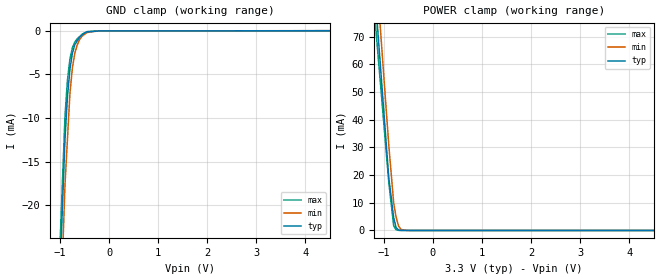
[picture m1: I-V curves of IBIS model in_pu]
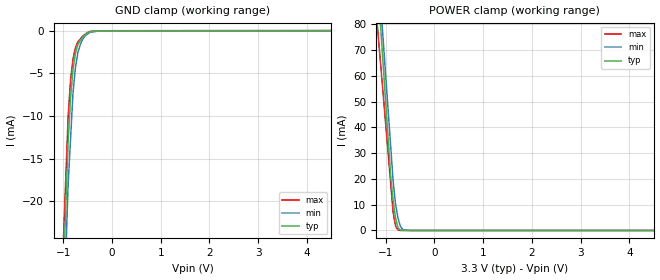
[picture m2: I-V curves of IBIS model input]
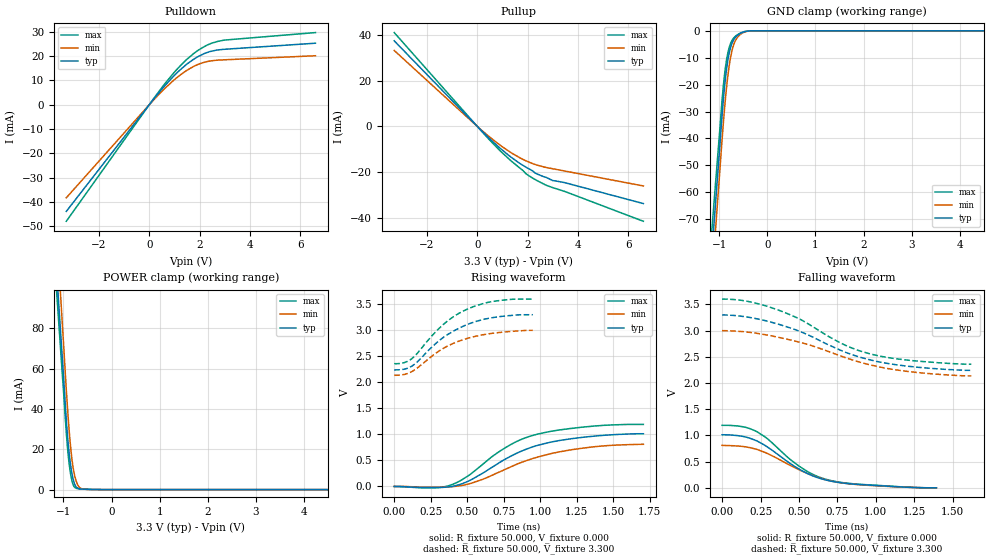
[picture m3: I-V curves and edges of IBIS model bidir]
|Texas Instruments Incorporated
|118dB SNR Stereo Audio ADC
[IBIS Ver]   4.0
[File Name] pcm4202.ibs
[File Rev] 3.0
[Date]   10-06-2009
[Notes]  Quality Check of this IBIS model: Model Passes IBIS Check. Model
   parses into ICX IS. Simulates with Hyperlynx.
   1. MIN TYP MAX information is based on Temperature and Voltage
   characteristics only.
   2. Package information extracted using Tektronix IConnect Software.
[Source]   Texas Instruments Incorporated.
   Analog-eLab, HPA
   12500 TI Blvd
   Dallas, TX -75243
   For Support e-mail: elab_ibis@list.ti.com
[Disclaimer]
| This model is designed as an aid for customers of Texas Instruments.
| TI and its licensors and suppliers make no warranties, either expressed
| or implied, with respect to this  model, including the warranties of
| merchantability or fitness for a particular purpose. The model is
| provided solely on an "as is" basis. The entire risk as to its quality
| and performance is with the customer.
[Copyright]
| (C) Copyright 2011 Texas Instruments Incorporated. All rights reserved.
[Component] PCM4202
[Manufacturer] TI
[Package]
| variable   typ   min   max
R_pkg  1.000E-02   1.000E-02   1.000E-02
L_pkg  2.970E-09   2.790E-09   3.150E-09
C_pkg  4.580E-13   1.880E-13   7.280E-13
[Pin] signal_name  model_name  R_pin  L_pin C_pin
1   VREFL   term   1.000E-02   3.150E-09   7.280E-13
2   AGNDL   GND   1.000E-02   3.090E-09   6.380E-13
3   VCOML   POWER   1.000E-02   3.030E-09   5.480E-13
4   VINL_P   term   1.000E-02   2.970E-09   4.580E-13
5   VINL_M   term   1.000E-02   2.910E-09   3.680E-13
6   FMT0   input   1.000E-02   2.850E-09   2.780E-13
7   FMT1   input   1.000E-02   2.790E-09   1.880E-13
8   S/*M   input   1.000E-02   2.790E-09   1.880E-13
9   OSR0   input   1.000E-02   2.850E-09   2.780E-13
10  OSR1   input   1.000E-02   2.910E-09   3.680E-13
11  OSR2   input   1.000E-02   2.970E-09   4.580E-13
12  BYPAS   input   1.000E-02   3.030E-09   5.480E-13
13  DGND   GND   1.000E-02   3.090E-09   6.380E-13
14  VDD   POWER   1.000E-02   3.150E-09   7.280E-13
15  DATA/DSDR   output  1.000E-02   3.150E-09   7.280E-13
16  BCK/DSDL   bidir   1.000E-02   3.090E-09   6.380E-13
17  LRCK/DSDBCK bidir   1.000E-02   3.030E-09   5.480E-13
18  SCKI   input   1.000E-02   2.970E-09   4.580E-13
19  *RST   in_pu   1.000E-02   2.910E-09   3.680E-13
20  CLIPR   output  1.000E-02   2.850E-09   2.780E-13
21  CLIPL   output  1.000E-02   2.790E-09   1.880E-13
22  VCC   POWER   1.000E-02   2.790E-09   1.880E-13
23  AGND   GND   1.000E-02   2.850E-09   2.780E-13
24  VINR_M   term   1.000E-02   2.910E-09   3.680E-13
25  VINR_P   term   1.000E-02   2.970E-09   4.580E-13
26  VCOMR   POWER   1.000E-02   3.030E-09   5.480E-13
27  AGNDR   GND   1.000E-02   3.090E-09   6.380E-13
28  VREFR   term   1.000E-02   3.150E-09   7.280E-13
[Diff Pin] inv_pin vdiff tdelay_typ tdelay_min tdelay_max
4  5   NA   NA  NA  NA
25 24  NA   NA  NA  NA
[Model]  term
Model_type Terminator
C_comp   0   0   0
[Voltage Range]  5.00  4.75  5.25
[Temperature Range] 25   70   -10
| Models and submodels in the file (5): in_pu (Input), input (Input), bidir (I/O), output (Output), term (Terminator)
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[Model] in_pu
Model_type Input
Vinl = 990.000mV
Vinh = 2.31000V
C_comp 886.000fF 877.000fF 891.000fF
| variable typ   min   max
[Voltage Range] 3.30000V 3.00000V 3.60000V
[POWER Clamp Reference] 3.30000V 3.00000V 3.60000V
[GND Clamp Reference] 0.00000V 0.00000V 0.00000V
[Temperature Range] 25   70   -10
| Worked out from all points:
|   GND clamp passes 1 mA (typ) near -0.63 V on its own axis
|   POWER clamp passes 1 mA (typ) near -0.75 V on its own axis
[GND Clamp]
-3.3V     -369.9mA   -412.4mA   -356.3mA
-900mV    -12.43mA   -17.61mA   -9.82mA
-850mV    -7.567mA   -12.41mA   -5.659mA
-800mV    -4.432mA   -7.205mA   -3.254mA
-750mV    -2.598mA   -4.295mA   -1.972mA
-700mV    -1.601mA   -2.555mA   -1.295mA
-650mV    -1.153mA   -1.615mA   -919.1uA
-600mV    -704.6uA   -986.7uA   -654.8uA
-550mV    -481.7uA   -601.4uA   -390.5uA
-450mV    -126.3uA   -189.9uA   -94.7uA
-225mV    -21.91uA   -16.78uA   -19.72uA
6.6V      22.46uA    24.13uA    17.33uA
[POWER Clamp]
-3.3V     589.8mA    621.3mA    521.2mA
-1.15V    78.61mA    92.45mA    70.07mA
-1.1V     66.72mA    80.15mA    59.58mA
-1.05V    54.83mA    67.86mA    49.09mA
-900mV    19.17mA    30.96mA    17.62mA
-800mV    4.66mA     10.03mA    1.697mA
-750mV    1.031mA    4.804mA    243.3uA
-700mV    165.1uA    1.618mA    31.19uA
-650mV    23.84uA    330.3uA    28.07uA
-550mV    16.51uA    39.34uA    21.83uA
6.6V      0A         0A         0A
[Model] input
Model_type Input
Vinl = 990.000mV
Vinh = 2.31000V
C_comp 696.000fF 674.000fF 706.000fF
| variable typ   min   max
[Voltage Range] 3.30000V 3.00000V 3.60000V
[POWER Clamp Reference] 3.30000V 3.00000V 3.60000V
[GND Clamp Reference] 0.00000V 0.00000V 0.00000V
[Temperature Range] 25   70   -10
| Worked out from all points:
|   GND clamp passes 1 mA (typ) near -0.63 V on its own axis
|   POWER clamp passes 1 mA (typ) near -0.75 V on its own axis
[GND Clamp]
-3.3V     -397.4mA   -428.1mA   -369.7mA
-900mV    -12.92mA   -18mA      -10.03mA
-850mV    -7.77mA    -12.64mA   -5.758mA
-800mV    -4.508mA   -7.277mA   -3.299mA
-750mV    -2.625mA   -4.318mA   -1.991mA
-700mV    -1.61mA    -2.56mA    -1.301mA
-650mV    -1.156mA   -1.614mA   -958.6uA
-600mV    -701.1uA   -983.5uA   -616.6uA
-550mV    -475.7uA   -595.5uA   -410uA
-450mV    -115.8uA   -182uA     -82.78uA
-225mV    -9.94uA    -7.128uA   -5.494uA
6.6V      10.56uA    13.27uA    6.381uA
[POWER Clamp]
-3.3V     700.9mA    675.4mA    555.4mA
-1.15V    91.83mA    99.8mA     74.4mA
-1.1V     77.66mA    86.41mA    63.21mA
-1.05V    63.5mA     73.02mA    52.02mA
-900mV    21mA       32.86mA    18.46mA
-850mV    11.63mA    19.48mA    7.275mA
-800mV    4.861mA    10.31mA    1.694mA
-750mV    1.037mA    4.862mA    240.6uA
-700mV    163.9uA    1.623mA    30.23uA
-650mV    24.11uA    329uA      27.21uA
-550mV    16.69uA    39.36uA    21.16uA
6.6V      0A         0A         0A
[Model]   bidir
Model_type I/O
Vinl=9.900E-01
Vinh=2.310E+00
Vref=0.000E+00
Rref=1.000E+06
Cref=1.500E-12
Vmeas=1.650E+00
C_comp   9.430E-13   9.350E-13   9.520E-13
[Voltage Range]   3.300E+00   3.000E+00   3.600E+00
[POWER Clamp Reference]   3.300E+00   3.000E+00   3.600E+00
[GND Clamp Reference]   0.000E+00   0.000E+00   0.000E+00
[Pullup Reference]   3.300E+00   3.000E+00   3.600E+00
[Pulldown Reference]   0.000E+00   0.000E+00   0.000E+00
[Temperature Range]   25   70   -10
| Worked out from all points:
|   slope of the pulldown table from 0 to 0.495 V, typ, clamps not added: 78.3 ohm
|   slope of the pullup table from 0 to 0.495 V, typ, clamps not added: 91.8 ohm
|   GND clamp passes 1 mA (typ) near -0.56 V on its own axis
|   POWER clamp passes 1 mA (typ) near -0.72 V on its own axis
|   rising waveform, R_fixture 50.000, V_fixture 0.000: 20-80 % time 437ps typ, 475ps min, 395ps max; typ from 0 V to 1.01 V
|   falling waveform, R_fixture 50.000, V_fixture 0.000: 20-80 % time 336ps typ, 365ps min, 317ps max; typ from 1.01 V to 0 V
|   rising waveform, R_fixture 50.000, V_fixture 3.300: 20-80 % time 301ps typ, 307ps min, 288ps max; typ from 2.24 V to 3.3 V
|   falling waveform, R_fixture 50.000, V_fixture 3.300: 20-80 % time 545ps typ, 586ps min, 502ps max; typ from 3.3 V to 2.24 V
[GND Clamp]
-3.3V     -594.8mA   -619.2mA   -559mA
-1.02V    -50.27mA   -59.71mA   -43.64mA
-940mV    -31.02mA   -39.98mA   -25.37mA
-900mV    -22.65mA   -30.92mA   -17.8mA
-860mV    -15.87mA   -23.04mA   -12.09mA
-800mV    -8.816mA   -13.78mA   -6.61mA
-760mV    -5.897mA   -9.384mA   -4.492mA
-700mV    -3.299mA   -5.147mA   -2.643mA
-640mV    -1.977mA   -2.907mA   -1.67mA
-540mV    -768uA     -1.05mA    -647.7uA
-340mV    0A         0A         0A
6.6V      0A         0A         0A
[Power Clamp]
-3.3V     891.7mA    975.1mA    843.7mA
-1.02V    63.8mA     80.91mA    55.99mA
-940mV    34.42mA    49.33mA    27.99mA
-900mV    22.41mA    35.18mA    16.83mA
-880mV    17.71mA    28.96mA    12.52mA
-840mV    10.45mA    18.55mA    6.172mA
-820mV    7.621mA    14.45mA    4.01mA
-780mV    3.552mA    8.365mA    1.558mA
-740mV    1.454mA    4.573mA    714.5uA
-660mV    404uA      925.2uA    318uA
-480mV    99.23uA    56.36uA    154uA
6.6V      0A         0A         0A
[Pullup]
-3.3V     37.41mA    33.19mA    41.01mA
380mV     -4.204mA   -3.617mA   -4.623mA
820mV     -8.717mA   -7.476mA   -9.668mA
1.28V     -12.92mA   -11.04mA   -14.44mA
1.82V     -17.05mA   -14.45mA   -19.31mA
1.92V     -17.72mA   -14.96mA   -20.56mA
2.2V      -19.44mA   -16.26mA   -22.59mA
2.3V      -20.41mA   -16.65mA   -23.22mA
2.74V     -22.3mA    -17.96mA   -25.71mA
3V        -23.67mA   -18.51mA   -26.77mA
3.46V     -24.54mA   -19.47mA   -28.35mA
6.6V      -33.73mA   -26.03mA   -41.47mA
[Pulldown]
-3.3V     -43.9mA    -38.31mA   -47.97mA
0V        0A         0A         0A
480mV     6.141mA    5.273mA    6.774mA
1.06V     12.71mA    10.84mA    14.11mA
1.46V     16.43mA    13.92mA    18.35mA
1.76V     18.67mA    15.71mA    21.01mA
2.28V     21.38mA    17.67mA    24.42mA
2.68V     22.44mA    18.27mA    25.9mA
2.98V     22.76mA    18.44mA    26.55mA
6.6V      25.27mA    20.11mA    29.64mA
[Rising Waveform]
R_fixture = 50.000
V_fixture = 0.000
V_fixture_min = 0.000
V_fixture_max = 0.000
|  time   V(typ)   V(min)   V(max)
0s        0V         0V         0V
262.5ps   -21.75mV   -13.38mV   -26.33mV
390ps     -1.601mV   -5.427mV   29.79mV
527.5ps   128.6mV    61.72mV    245.9mV
675ps     376.9mV    220.7mV    583.2mV
762.5ps   527.7mV    330.8mV    746.5mV
870ps     676.7mV    461.1mV    902.8mV
992.5ps   797.9mV    572.2mV    1.013V
1.343ns   959.6mV    753.7mV    1.154V
1.707ns   1.013V     810.4mV    1.193V
[Falling Waveform]
R_fixture = 50.000
V_fixture = 0.000
V_fixture_min = 0.000
V_fixture_max = 0.000
|  time   V(typ)   V(min)   V(max)
0s        1.013V     810.4mV    1.193V
130ps     983.9mV    790.8mV    1.168V
220ps     903.5mV    738.9mV    1.081V
292.5ps   784.4mV    658.2mV    942.5mV
422.5ps   507.3mV    460.4mV    593.5mV
497.5ps   363.5mV    350.2mV    421.5mV
590ps     229.3mV    234.1mV    257.8mV
667.5ps   155.8mV    160.3mV    170.3mV
895ps     63.2mV     59.31mV    67.64mV
1.395ns   0V         0V         0V
[Rising Waveform]
R_fixture = 50.000
V_fixture = 3.300
V_fixture_min = 3.000
V_fixture_max = 3.600
|  time   V(typ)   V(min)   V(max)
0s        2.241V     2.136V     2.358V
65ps      2.252V     2.151V     2.377V
117.5ps   2.307V     2.202V     2.449V
332.5ps   2.856V     2.647V     3.104V
410ps     2.991V     2.756V     3.27V
487.5ps   3.097V     2.834V     3.391V
597.5ps   3.2V       2.909V     3.505V
677.5ps   3.246V     2.946V     3.556V
812.5ps   3.289V     2.982V     3.598V
950ps     3.3V       3V         3.6V
[Falling Waveform]
R_fixture = 50.000
V_fixture = 3.300
V_fixture_min = 3.000
V_fixture_max = 3.600
|  time   V(typ)   V(min)   V(max)
0s        3.3V       3V         3.6V
172.5ps   3.254V     2.968V     3.554V
385ps     3.105V     2.86V      3.371V
507.5ps   2.983V     2.775V     3.216V
770ps     2.626V     2.518V     2.765V
882.5ps   2.506V     2.409V     2.626V
965ps     2.44V      2.345V     2.554V
1.08ns    2.372V     2.275V     2.485V
1.267ns   2.303V     2.201V     2.419V
1.622ns   2.241V     2.136V     2.358V
[Ramp]
dV/dt_r   6.1203E-01/4.3463E-10   4.8646E-01/4.7340E-10   7.1644E-01/3.9500E-10
dV/dt_f   6.3545E-01/5.4359E-10   5.1832E-01/5.8531E-10   7.4517E-01/5.0150E-10
R_load = 50
